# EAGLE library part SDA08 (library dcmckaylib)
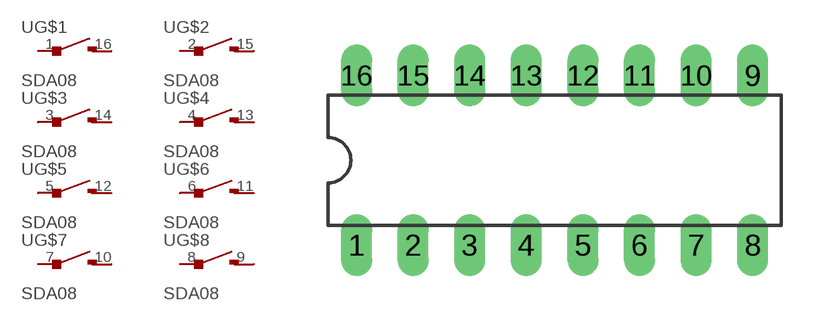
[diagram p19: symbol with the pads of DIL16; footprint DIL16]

Designator prefix -; gates G$1=SPSTSWITCH2 G$2=SPSTSWITCH2 G$3=SPSTSWITCH2 G$4=SPSTSWITCH2 G$5=SPSTSWITCH2 G$6=SPSTSWITCH2 G$7=SPSTSWITCH2 G$8=SPSTSWITCH2

## SDA08  [DIL16]
1  G$1:P$1
2  G$2:P$1
3  G$3:P$1
4  G$4:P$1
5  G$5:P$1
6  G$6:P$1
7  G$7:P$1
8  G$8:P$1
9  G$8:P$3
10  G$7:P$3
11  G$6:P$3
12  G$5:P$3
13  G$4:P$3
14  G$3:P$3
15  G$2:P$3
16  G$1:P$3

## Footprint DIL16 (pad centres in mm)
Dual In Line Package
drill 0.889 long: 1 -8.89,-3.81; 2 -6.35,-3.81; 3 -3.81,-3.81; 4 -1.27,-3.81; 5 1.27,-3.81; 6 3.81,-3.81; 7 6.35,-3.81; 8 8.89,-3.81; 9 8.89,3.81; 10 6.35,3.81; 11 3.81,3.81; 12 1.27,3.81; 13 -1.27,3.81; 14 -3.81,3.81; 15 -6.35,3.81; 16 -8.89,3.81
